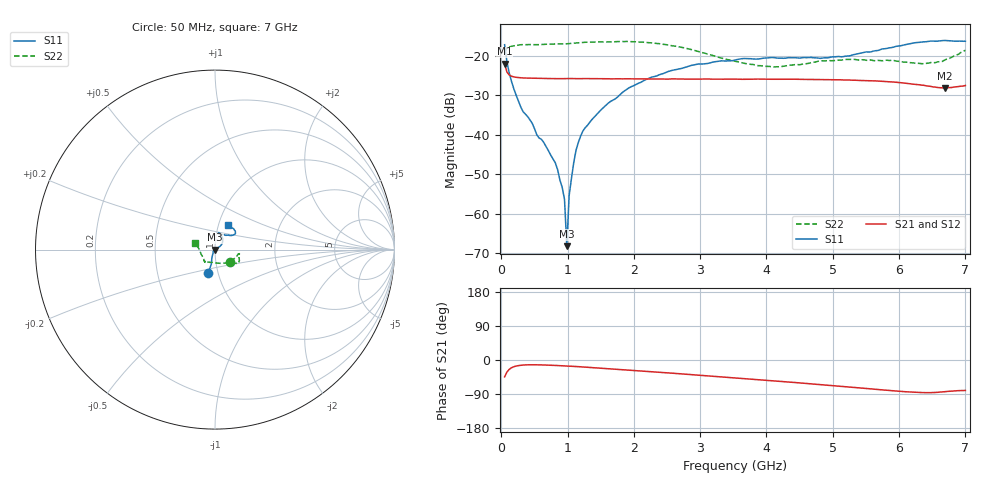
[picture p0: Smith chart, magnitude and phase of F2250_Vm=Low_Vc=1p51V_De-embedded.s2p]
! Integrated Device Technology
! Corporate Headquarters
! 6024 Silver Creek Valley Road
! San Jose, CA 95138  USA
! Phone:  1-408-284-8200
! Toll Free:  1-800-223-1366
! Webpage:  http://www.idt.com/
! Timing and RF Division
! 515 Groton Road, Suite 102
! Westford, MA 01886-6024
! Device:  F2250
! Description: Voltage Variable RF Attenuator
! Frequency:  50.0 -  6000.00 MHz
! Package:  3x3 mm Thin QFN Plastic Package: 16 pin
! Ports:  2 RF, 3 DC
!  Pin  1  = GND
!  Pin  2  = NC
!  Pin  3  = RF1  = Port 1
!  Pin  4  = NC
!  Pin  5  = GND
!  Pin  6  = GND
!  Pin  7  = GND
!  Pin  8  = GND
!  Pin  9  = NC
!  Pin 10  = RF2  = Port 2
!  Pin 11  = NC
!  Pin 12  = GND
!  Pin 13  = GND
!  Pin 14  = VCNTRL
!  Pin 15  = VDD
!  Pin 16  = VMODE
! Vcntrl:  1.510 Volts
! Vmode:  +0.000 Volts
! Vdd:  +3.30  Volts
! Current:  1.191 mA
! Data:  The device was measured on a the F2250 evaluation board which has
!  individual transmission lines to the RF pins.  Data was collected
!  using a calibrated network analyzer.  The evaluation board was
!  de-embedded using a TRL calibration technique.
!  The reference plane is the edge of the package pin.
! Misc:  SN 10
!  Action Tracker AT0258
! Date Measured:  2014-11-26
! Date:  2015-10-15  MJV
! Note:
!  Integrated Device Technology supplies this data as a sample of measured
!  data at the package pin for this product.  Your particular data for this
!  product may vary.
!  Data was taken at 25 degrees C.
!  Integrated Device Technology reserves the right to change this data at anytime.
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# GHz S dB R 50
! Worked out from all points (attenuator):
!   201 points, 50 MHz to 7 GHz, reference 50 ohm
!   highest |S21| = -22.01 dB at 50 MHz (marker M1); lowest = -28.2 dB at 6.687 GHz (marker M2)
!   lowest |S11| = -68.2 dB at 988.2 MHz (marker M3), VSWR 1.00, Z = 50 - j0.00868 ohm
!   |S11| at or under -10 dB: start of sweep to end of sweep
!   |S22| runs from -22.8 to -16.4 dB; largest |S21 - S12| = 0.00021
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0.05  -17.22 -106.4  -22.01 -44.6  -22.00 -44.6  -19.27 -38.2
0.1195  -24.37 -107.5  -24.86 -24.6  -24.84 -24.6  -17.76 -13.1
0.29325  -32.95 -117.8  -25.59 -13.9  -25.60 -13.9  -17.23 -10.0
0.64075  -41.95 -144.0  -25.75 -13.1  -25.74 -13.1  -17.13 -13.3
0.84925  -48.79 178.4  -25.80 -14.6  -25.81 -14.6  -17.02 -17.2
0.9535  -56.34 -165.0  -25.79 -15.5  -25.80 -15.5  -17.06 -18.9
0.98825  -68.18 -12.8  -25.79 -15.8  -25.81 -15.8  -16.98 -19.3
1.023  -55.42 11.1  -25.79 -16.2  -25.79 -16.2  -16.94 -19.5
1.05775  -51.10 18.4  -25.78 -16.5  -25.79 -16.5  -16.91 -19.9
1.12725  -43.92 21.4  -25.81 -17.2  -25.82 -17.2  -16.79 -21.1
1.2315  -39.02 22.9  -25.81 -18.3  -25.80 -18.4  -16.65 -22.9
1.5095  -33.60 28.8  -25.82 -21.7  -25.83 -21.7  -16.53 -25.3
1.857  -28.92 33.8  -25.84 -25.9  -25.82 -25.9  -16.42 -28.7
2.37825  -24.86 43.0  -25.89 -32.3  -25.88 -32.3  -16.94 -32.8
2.93425  -22.21 57.1  -25.92 -39.3  -25.90 -39.3  -18.76 -40.7
3.525  -21.10 70.5  -25.93 -47.1  -25.92 -47.1  -21.40 -64.4
4.11575  -20.49 78.5  -25.96 -55.0  -25.96 -55.0  -22.85 -97.3
4.7065  -20.52 71.3  -26.01 -63.4  -26.01 -63.4  -21.67 -120.8
5.85325  -18.02 39.4  -26.61 -80.4  -26.58 -80.5  -21.22 -134.5
6.3745  -16.49 40.6  -27.49 -86.1  -27.52 -86.1  -22.02 -154.6
6.68725  -16.14 48.1  -28.17 -83.6  -28.13 -83.7  -21.11 178.4
7  -16.34 62.8  -27.55 -80.3  -27.54 -80.4  -18.63 163.0
